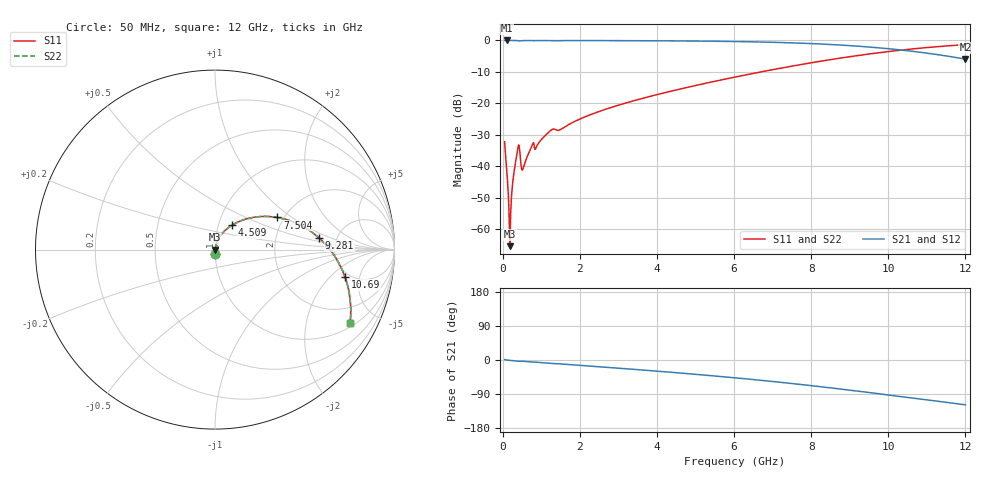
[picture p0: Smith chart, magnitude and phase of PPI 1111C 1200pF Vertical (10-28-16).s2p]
# GHz S MA R 50
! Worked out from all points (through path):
!   1601 points, 50 MHz to 12 GHz, reference 50 ohm
!   highest |S21| = 0.00 dB at 102.3 MHz (marker M1); lowest = -5.9 dB at 12 GHz (marker M2)
!   group delay of S21, straight-line fit = 27.2 ps
!   lowest |S11| = -65.4 dB at 184.4 MHz (marker M3), VSWR 1.00, Z = 50.1 - j0.0129 ohm
!   |S11| at or under -10 dB: start of sweep to 6.698 GHz
!   |S22| runs from -65.4 to -1.3 dB; largest |S21 - S12| = 0
!   S11 on the Smith chart (normalised r, x): 50 MHz: 1.00, -0.05; 4.509 GHz: 1.16, +0.32; 7.504 GHz: 1.85, +0.78; 9.281 GHz: 3.65, +0.72; 10.69 GHz: 4.56, -3.07; 12 GHz: 1.15, -3.57
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0.05  0.02446 -88.1  0.9994 1.1  0.9994 1.1  0.02446 -88.1
0.1022813  0.009096 -87.5  0.9996 -0.0  0.9996 -0.0  0.009096 -87.5
0.139625  0.004242 -84.4  0.9995 -0.5  0.9995 -0.5  0.004242 -84.4
0.1844375  0.0005374 -13.8  0.9995 -1.0  0.9995 -1.0  0.0005374 -13.8
0.2217813  0.002782 76.0  0.9994 -1.4  0.9994 -1.4  0.002782 76.0
0.2964688  0.008259 80.6  0.9989 -2.1  0.9989 -2.1  0.008259 80.6
0.3562187  0.01411 75.4  0.997 -2.7  0.997 -2.7  0.01411 75.4
0.3935625  0.01958 62.3  0.9917 -3.2  0.9917 -3.2  0.01958 62.3
0.5354688  0.00941 58.9  0.9956 -3.4  0.9956 -3.4  0.00941 58.9
0.7520625  0.0205 76.5  0.9968 -5.3  0.9968 -5.3  0.0205 76.5
0.8790313  0.02065 76.2  0.9969 -6.0  0.9969 -6.0  0.02065 76.2
1.222594  0.03611 74.9  0.9953 -8.7  0.9953 -8.7  0.03611 74.9
2.044156  0.05782 73.1  0.9957 -14.4  0.9957 -14.4  0.05782 73.1
4.038312  0.1395 59.2  0.9872 -29.7  0.9872 -29.7  0.1395 59.2
4.508844  0.1639 55.4  0.9833 -33.6  0.9833 -33.6  0.1639 55.4
6.025  0.2618 42.2  0.9612 -47.0  0.9612 -47.0  0.2618 42.2
7.503813  0.3907 27.3  0.9156 -62.1  0.9156 -62.1  0.3907 27.3
8.019156  0.4433 21.5  0.891 -67.8  0.891 -67.8  0.4433 21.5
9.281375  0.5837 6.4  0.8054 -83.1  0.8054 -83.1  0.5837 6.4
10.01331  0.6669 -3.0  0.7379 -92.4  0.7379 -92.4  0.6669 -3.0
10.69297  0.7401 -11.9  0.6645 -101.3  0.6645 -101.3  0.7401 -11.9
12  0.8573 -28.7  0.5052 -118.1  0.5052 -118.1  0.8573 -28.7
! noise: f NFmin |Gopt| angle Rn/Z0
0.05  0.0003799  0.8686  0.2867  0.0006219
1.372  0.0107  0.8722  7.447  0.01797
2.701  0.007843  0.6929  14.3  0.004903
4.031  0.01024  0.6615  20.95  0.005605
5.36  0.01289  0.6527  27.32  0.006685
6.682  0.0159  0.6584  33.38  0.008185
8.012  0.01957  0.6758  39.24  0.01038
9.341  0.02426  0.7033  44.91  0.01377
10.67  0.03065  0.7397  50.46  0.01939
12  0.04007  0.7835  55.98  0.02975
